FUNCTION FC 11 : VOID
TITLE =COMANDI PROFIBUS AZIONAMENTO 11 PROFILA 9 (SLAVE 8)
VERSION : 0.1

BEGIN
NETWORK
TITLE =TRASFERISCO I SEGNALI DI COMANDO
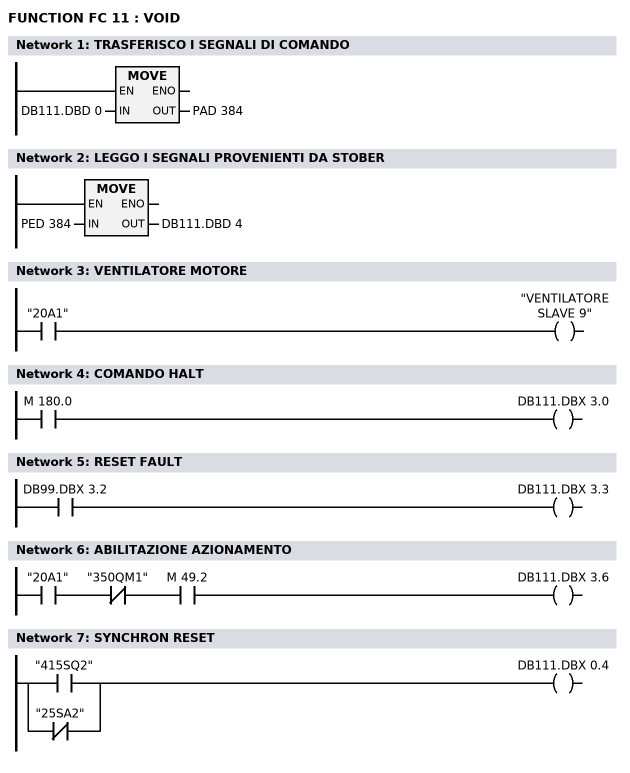
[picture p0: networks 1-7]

      L     DB111.DBD    0;
      T     PAD  384;
      NOP   0;
NETWORK
TITLE =LEGGO I SEGNALI PROVENIENTI DA STOBER

      L     PED  384;
      T     DB111.DBD    4;
      NOP   0;
NETWORK
TITLE =VENTILATORE MOTORE

      U     "20A1";
      =     "VENTILATORE SLAVE 9";
NETWORK
TITLE =COMANDO HALT

      U     M    180.0;
      =     DB111.DBX    3.0;
NETWORK
TITLE =RESET FAULT

      U     DB99.DBX    3.2;
      =     DB111.DBX    3.3;
NETWORK
TITLE =ABILITAZIONE AZIONAMENTO

      U     "20A1";
      UN    "350QM1";
      U     M     49.2;
      =     DB111.DBX    3.6;
NETWORK
TITLE =SYNCHRON RESET

      O     "415SQ2";
      ON    "25SA2";
      =     DB111.DBX    0.4;
END_FUNCTION

